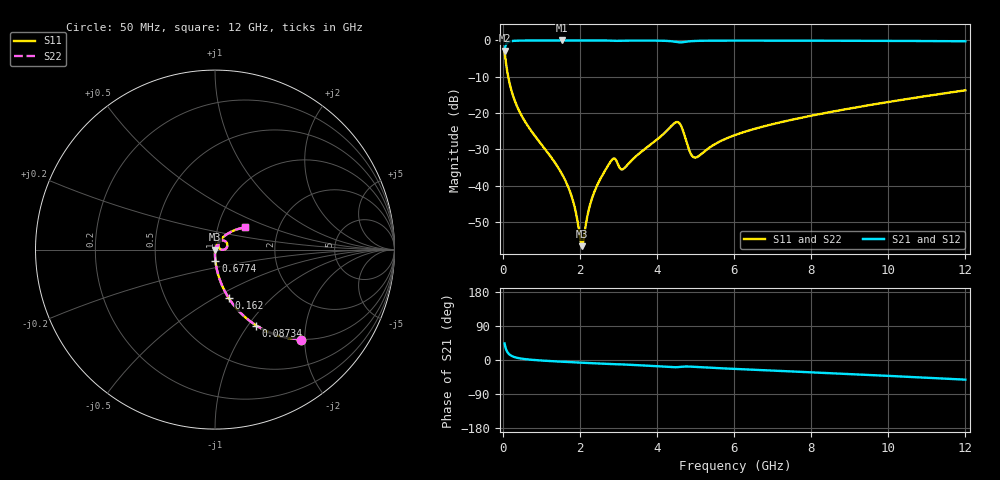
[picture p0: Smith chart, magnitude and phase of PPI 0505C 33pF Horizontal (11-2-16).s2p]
# MHz S MA R 50
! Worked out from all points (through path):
!   1601 points, 50 MHz to 12 GHz, reference 50 ohm
!   highest |S21| = -0.01 dB at 1.529 GHz (marker M1); lowest = -2.8 dB at 50 MHz (marker M2)
!   group delay of S21, straight-line fit = 13 ps
!   lowest |S11| = -56.6 dB at 2.052 GHz (marker M3), VSWR 1.00, Z = 50.1 - j0.031 ohm
!   |S11| at or under -10 dB: 143.5 MHz to end of sweep
!   |S22| runs from -56.6 to -3.2 dB; largest |S21 - S12| = 0
!   S11 on the Smith chart (normalised r, x): 50 MHz: 0.99, -1.92; 87.34 MHz: 0.99, -1.10; 162 MHz: 1.00, -0.59; 677.4 MHz: 1.00, -0.13; 12 GHz: 1.34, +0.35
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50  0.6925 -46.3  0.7212 43.7  0.7212 43.7  0.6925 -46.3
87.34375  0.4812 -61.5  0.8763 28.5  0.8763 28.5  0.4812 -61.5
162.0312  0.2826 -74.1  0.9588 15.9  0.9588 15.9  0.2826 -74.1
356.2188  0.1299 -83.5  0.9909 6.2  0.9909 6.2  0.1299 -83.5
677.375  0.0636 -88.0  0.9971 1.3  0.9971 1.3  0.0636 -88.0
1528.812  0.01481 -89.8  0.9986 -4.5  0.9986 -4.5  0.01481 -89.8
1812.625  0.006509 -84.1  0.9985 -5.9  0.9985 -5.9  0.006509 -84.1
2044.156  0.001502 -19.2  0.9984 -7.1  0.9984 -7.1  0.001502 -19.2
2051.625  0.001479 -12.1  0.9984 -7.1  0.9984 -7.1  0.001479 -12.1
2350.375  0.007571 67.6  0.998 -8.6  0.998 -8.6  0.007571 67.6
2798.5  0.02154 61.1  0.993 -10.9  0.993 -10.9  0.02154 61.1
2903.062  0.02368 47.4  0.9873 -11.2  0.9873 -11.2  0.02368 47.4
3127.125  0.01705 54.7  0.9929 -11.7  0.9929 -11.7  0.01705 54.7
4038.312  0.04485 64.9  0.9921 -16.5  0.9921 -16.5  0.04485 64.9
4546.188  0.07513 25.7  0.9446 -18.7  0.9446 -18.7  0.07513 25.7
4650.75  0.06239 6.2  0.9423 -17.5  0.9423 -17.5  0.06239 6.2
4874.812  0.02778 9.1  0.9748 -17.5  0.9748 -17.5  0.02778 9.1
5001.781  0.02447 30.5  0.9834 -18.3  0.9834 -18.3  0.02447 30.5
6025  0.0499 61.1  0.9937 -23.5  0.9937 -23.5  0.0499 61.1
8019.156  0.09246 55.1  0.9915 -32.6  0.9915 -32.6  0.09246 55.1
10013.31  0.1426 46.4  0.9851 -42.0  0.9851 -42.0  0.1426 46.4
12000  0.2059 36.8  0.9732 -51.9  0.9732 -51.9  0.2059 36.8
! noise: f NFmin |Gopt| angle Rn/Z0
50  0.0003895  0.8652  0.755  0.0006203
1372  0.004002  0.6753  4.862  0.002373
2701  0.01033  0.7431  9.329  0.008016
4031  0.01629  0.7563  13.84  0.01332
5360  0.02039  0.7447  18.38  0.01564
6682  0.01648  0.6345  22.51  0.008177
8012  0.01754  0.601  26.58  0.007702
9341  0.01932  0.5867  30.55  0.007988
1.067e+04  0.02139  0.581  34.41  0.008537
1.2e+04  0.02367  0.5808  38.14  0.009255
